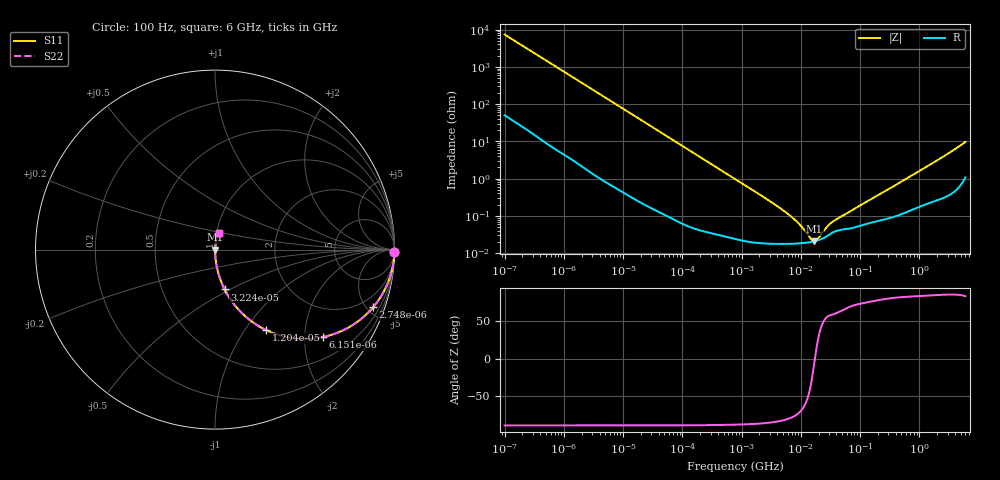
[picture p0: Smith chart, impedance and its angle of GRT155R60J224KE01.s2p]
!Murata Part Number: GRT155R60J224KE01
!These Parameters are Measured in Series Mode Connection
!Data Generated on Jun 19, 2026
!  o--ll--o
!Port1  Port2
!  o------o
!Operation Temp=25[degC], DC Bias Voltage=0[V]
!Freq. Start=100[Hz] Stop=6[GHz] 401[Steps]
# Hz S RI R 50
!Freq.(Hz) S11(Real) S11(Imag) S21(Real) S21(Imag) S12(Real) S12(Imag) S22(Real) S22(Imag)
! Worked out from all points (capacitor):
!   401 points, 100 Hz to 6 GHz, reference 50 ohm
!   read as one part in series: C = 214 nF near 109 Hz
!   lowest |Z| = 21 mohm at 17.01 MHz (marker M1)
!   series resonance near 17.31 MHz, so ESL is about 390 pH
!   S11 on the Smith chart (normalised r, x): 100 Hz: open; 2.748 kHz: 1.03, -5.47; 6.151 kHz: 1.01, -2.45; 12.04 kHz: 1.01, -1.25; 32.24 kHz: 1.00, -0.47; 6 GHz: 1.02, +0.19
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100  0.9997 -0.0135  0.000274 0.0135  0.000274 0.0135  0.9997 -0.0135
600  0.9931 -0.0797  0.00687 0.0797  0.00687 0.0797  0.9931 -0.0797
2008  0.9319 -0.2491  0.0681 0.2491  0.0681 0.2491  0.9319 -0.2491
2748  0.8805 -0.3216  0.1195 0.3216  0.1195 0.3216  0.8805 -0.3216
4111  0.7686 -0.4191  0.2314 0.4191  0.2314 0.4191  0.7686 -0.4191
6151  0.599 -0.4874  0.401 0.4874  0.401 0.4874  0.599 -0.4874
12041  0.283 -0.4476  0.717 0.4476  0.717 0.4476  0.283 -0.4476
18841  0.14 -0.344  0.86 0.344  0.86 0.344  0.14 -0.344
32244  0.0535 -0.2218  0.9465 0.2218  0.9465 0.2218  0.0535 -0.2218
40335  0.0352 -0.181  0.9648 0.181  0.9648 0.181  0.0352 -0.181
129199  0.00397 -0.0586  0.996 0.0586  0.996 0.0586  0.00397 -0.0586
774597  0.000337 -0.00988  0.9997 0.00988  0.9997 0.00988  0.000337 -0.00988
6075234  0.000179 -0.00111  0.9998 0.00111  0.9998 0.00111  0.000179 -0.00111
9506416  0.000184 -0.000566  0.9998 0.000566  0.9998 0.000566  0.000184 -0.000566
1.555665e7  0.000203 -9.48e-05  0.9998 9.48e-05  0.9998 9.48e-05  0.000203 -9.48e-05
1.701401e7  0.000209 -1.5e-05  0.9998 1.5e-05  0.9998 1.5e-05  0.000209 -1.5e-05
1.946e7  0.000222 0.000104  0.9998 -0.000104  0.9998 -0.000104  0.000222 0.000104
2.784235e7  0.000289 0.000427  0.9997 -0.000427  0.9997 -0.000427  0.000289 0.000427
3.482834e7  0.000363 0.000608  0.9996 -0.000608  0.9996 -0.000608  0.000363 0.000608
3.124326e8  0.0009 0.0053  0.9991 -0.0053  0.9991 -0.0053  0.0009 0.0053
1.95892e9  0.00348 0.0301  0.9965 -0.0301  0.9965 -0.0301  0.00348 0.0301
6e9  0.0196 0.0934  0.9804 -0.0934  0.9804 -0.0934  0.0196 0.0934
